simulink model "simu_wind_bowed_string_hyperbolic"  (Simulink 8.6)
settings: Solver=ode4  StartTime=0.0  StopTime=runtime  FixedStep=1/fs  RelTol=1e-3
PostLoadFcn:
  | , if any(exist('dsrtsu_mdlpostloadfcn', 'file') == [2, 3, 6]), try dsrtsu_mdlpostloadfcn('Execute', bdroot); catch fprintf('Error in PostLoadFcn (dsrtsu_mdlpostloadfcn) for model "%s":
  |  %s
  | ', bdroot, lasterr); end, end,
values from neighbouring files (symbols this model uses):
  alpha = 0.5    [bowed_string_hyperbolic.m]    (also in polynomial.m = 100)
  an = modal_coeff(:,1)    [hybrid_wind.m]
  delta = mu_d/mu_s    (= 0.375)    [bowed_string_hyperbolic.m]
  gammab_cte = 1    [bowed_string_hyperbolic.m]
  PM = 50    [bowed_string_hyperbolic.m]    (also in lip_reed.m = 20; single_reed.m = 100)
  Qn = modal_coeff(:,3)    [hybrid_wind.m]
  Ts = 25e-6    (= 2.5e-05)    [hybrid_wind.m]    (also in measurements.m)
  wn = modal_coeff(:,2)    [hybrid_wind.m]
  Zc = rho*c/St    (= 2615281.00417)    [hybrid_wind.m]
  zetab_cte = 0.2    [bowed_string_hyperbolic.m]
undefined symbols (not defined in the file or in its folder): modal_coeff, vibrato
libraries: simulink x4

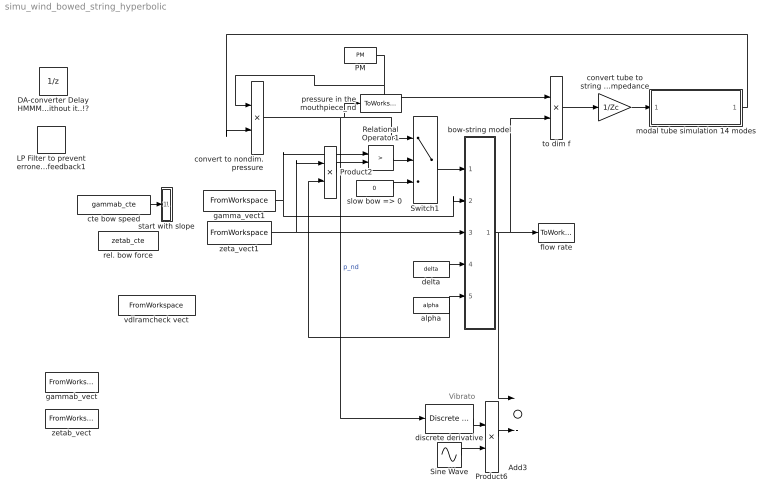
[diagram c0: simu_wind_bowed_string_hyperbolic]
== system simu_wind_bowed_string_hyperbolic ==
  note: Vibrato
  Add3 : Sum
  DA-converter Delay HMMM I don't know why this causes a less hybrid-corresponding result than without it..!? : UnitDelay  SampleTime=-1
  LP Filter to prevent erroneous high freq feedback1 : DiscreteFilter  Numerator=HdLP.ScaleValues(1)*HdLP.sosMatrix(1:end/2)  Denominator=HdLP.ScaleValues(2)*HdLP.sosMatrix(1+end/2:end)  SampleTime=Ts
  PM : Constant  Value=PM
  Product2 : Product  SampleTime=Ts
  Product6 : Product
  Relational Operator1 : RelationalOperator  Operator=>  OutDataTypeStr=boolean  SampleTime=Ts
  Sine Wave : Sin  Amplitude=vibrato.amp  Bias=-vibrato.amp  Frequency=vibrato.freq*2*pi  SampleTime=0
  Switch1 : Switch  Criteria=u2 > Threshold
  alpha : Constant  Value=alpha
  bow-string model : Subsystem
  convert tube to string characteristic impedance : Gain  Gain=1/Zc
  convert to nondim. pressure : Product  Inputs=/*
  cte bow speed : Constant  Value=gammab_cte
  delta : Constant  Value=delta
  discrete derivative : simulink/Discrete/Discrete Derivative  gainval=1.0  ICPrevScaledInput=0.0  InputProcessing=Inherited  OutMin=[]  OutMax=[]  OutDataType=fixdt(1, 16)  OutScaling=2^-10  DoSatur=off
  flow rate : ToWorkspace  VariableName=q_dl  SaveFormat=Structure  SampleTime=-1
  gamma_vect1 : FromWorkspace  VariableName=gammab_envs_all  SampleTime=0
  gammab_vect : FromWorkspace  VariableName=gammab_vect  SampleTime=Ts  OutputAfterFinalValue=Setting to zero
  modal tube simulation 14 modes : Subsystem
  pressure in the mouthpiece_nd : ToWorkspace  VariableName=p_dl  SaveFormat=Structure  SampleTime=-1
  rel. bow force : Constant  Value=zetab_cte
  slow bow => 0 : Constant  Value=0
  start with slope : Subsystem
  to dim f : Product
  vdlramcheck vect : FromWorkspace  VariableName=gammabrampcheck_vect  SampleTime=Ts  OutputAfterFinalValue=Setting to zero
  zeta_vect1 : FromWorkspace  VariableName=zetab_envs_all  SampleTime=0  OutputAfterFinalValue=Setting to zero
  zetab_vect : FromWorkspace  VariableName=zetab_vect  SampleTime=Ts  OutputAfterFinalValue=Setting to zero
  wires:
  PM/1 -> to dim f/1, convert to nondim. pressure/1
  modal tube simulation 14 modes/1(p_sim_out) -> convert to nondim. pressure/2
  delta/1 -> bow-string model/4(deltab)
  convert tube to string characteristic impedance/1 -> modal tube simulation 14 modes/1(flowrate_in)
  bow-string model/1(f) -> flow rate/1, to dim f/2, Add3/1
  to dim f/1 -> convert tube to string characteristic impedance/1
  cte bow speed/1 -> start with slope/1(gamma_in)
  convert to nondim. pressure/1 -> Switch1/1, pressure in the mouthpiece_nd/1, discrete derivative/1  "p_nd"
  discrete derivative/1 -> Product6/1
  Sine Wave/1 -> Product6/2
  Add3/1 -> ?  "new fdl"
  Product6/1 -> Add3/2
  alpha/1 -> Product2/2, bow-string model/5(alpha)
  zeta_vect1/1 -> bow-string model/3(zetab), Product2/1
  Relational Operator1/1 -> Switch1/2
  slow bow => 0/1 -> Switch1/3
  Switch1/1 -> bow-string model/1(vdl)
  Product2/1 -> Relational Operator1/2
  gamma_vect1/1 -> bow-string model/2(vbdl), Relational Operator1/1

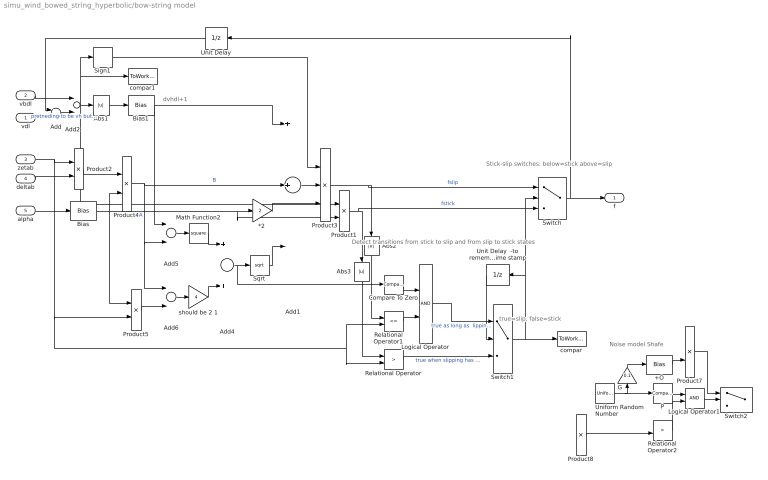
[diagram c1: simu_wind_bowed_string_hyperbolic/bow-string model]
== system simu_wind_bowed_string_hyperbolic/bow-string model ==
  note: Stick-slip switches: below=stick above=slip
  note: true=slip, false=stick
  note: dvhdl+1
  note: Detect transitions from stick to slip and from slip to stick states
  note: Noise model Shafe
  vdl : Inport
  vbdl : Inport  Port=2
  zetab : Inport  Port=3
  deltab : Inport  Port=4
  alpha : Inport  Port=5
  "*2 " : Gain  Gain=2
  +O : Bias  Bias=1
  Abs1 : Abs
  Abs2 : Abs
  Abs3 : Abs
  Add : Sum  Inputs=-+
  Add1 : Sum  Inputs=++-
  Add2 : Sum  Inputs=+-
  Add4 : Sum
  Add5 : Sum  Inputs=+-
  Add6 : Sum  Inputs=+-
  Bias : Bias  Bias=1
  Bias1 : Bias  Bias=1
  Compare To Zero : simulink/Logic and Bit Operations/Compare To Zero  relop=>  OutDataTypeStr=uint8
  G : Gain  Gain=0.1
  Logical Operator : Logic  AllPortsSameDT=off  OutDataTypeStr=boolean
  Logical Operator1 : Logic  AllPortsSameDT=off  OutDataTypeStr=boolean
  Math Function2 : Math  Operator=square
  P : simulink/Logic and Bit Operations/Compare To Constant  relop=>  const=0.5  OutDataTypeStr=uint8
  Product1 : Product  Inputs=*/
  Product{2,4..5,7..8} (5 alike) : Product
  Product3 : Product  Inputs=**/
  Relational Operator : RelationalOperator  Operator=>  OutDataTypeStr=boolean
  Relational Operator1 : RelationalOperator  Operator=<=  OutDataTypeStr=boolean
  Relational Operator2 : RelationalOperator  Operator=>  OutDataTypeStr=boolean
  Sign1 : Signum
  Sqrt : Sqrt  OutputSignalType=real
  Switch : Switch  Criteria=u2 > Threshold
  Switch1 : Switch  Criteria=u2 > Threshold
  Switch2 : Switch  Criteria=u2 > Threshold
  Uniform Random Number : UniformRandomNumber  Minimum=0  SampleTime=Ts
  Unit Delay : UnitDelay  SampleTime=-1
  Unit Delay  -to remember slip/stick state of previous time stamp : UnitDelay  SampleTime=-1
  compar : ToWorkspace  VariableName=compar  SaveFormat=Structure  SampleTime=-1
  compar1 : ToWorkspace  VariableName=dvhdl  SaveFormat=Structure  SampleTime=-1
  should be 2 1 : Gain  Gain=4
  f : Outport
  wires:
  vbdl/1 -> Add2/1
  Switch1/1 -> Switch/2, Unit Delay  -to remember slip/stick state of previous time stamp/1, compar/1
  Unit Delay  -to remember slip/stick state of previous time stamp/1 -> Switch1/2
  Add2/1 -> Abs1/1, Product1/1, Sign1/1, compar1/1
  Relational Operator/1 -> Switch1/3  "true when slipping has to start"
  Unit Delay/1 -> Add/1
  Add/1 -> Add2/2  "pretneding to be vh but is actually vh-1"
  vdl/1 -> Add/2
  Logical Operator/1 -> Switch1/1  "true as long as  lipping is happening"
  zetab/1 -> Product2/1, Product5/2, Relational Operator1/2, Relational Operator/2
  deltab/1 -> Product2/2
  Product2/1 -> Product4/1
  alpha/1 -> Bias/1
  Bias/1 -> Product1/2, "*2 "/1, Product5/1, Product4/2  "A"
  Product4/1 -> Add1/2, Add5/2, Add6/1  "B"
  Bias1/1 -> Add1/1, Add5/1
  Sqrt/1 -> Add1/3
  Add4/1 -> Sqrt/1, Compare To Zero/1
  Math Function2/1 -> Add4/1
  Add6/1 -> should be 2 1/1
  Add5/1 -> Math Function2/1
  should be 2 1/1 -> Add4/2
  Product5/1 -> Add6/2
  Abs1/1 -> Bias1/1
  Sign1/1 -> Product3/1
  Add1/1 -> Product3/2
  "*2 "/1 -> Product3/3
  Product1/1 -> Switch/3, Abs3/1  "fstick"
  Product3/1 -> Switch/1, Abs2/1  "fslip"
  Compare To Zero/1 -> Logical Operator/1
  Relational Operator1/1 -> Logical Operator/2
  Switch/1 -> Unit Delay/1, f/1
  Abs2/1 -> Relational Operator1/1
  Abs3/1 -> Relational Operator/1
  Logical Operator1/1 -> Switch2/2
  P/1 -> Logical Operator1/1
  Relational Operator2/1 -> Logical Operator1/2
  Uniform Random Number/1 -> P/1, G/1
  G/1 -> +O/1
  +O/1 -> Product7/2
  Product7/1 -> Switch2/1
  ? -> Relational Operator2/1  "dvhdl"
  Product8/1 -> Relational Operator2/2
  ? -> Product8/1  "1+alpha"
  ? -> Product8/2  "zetab"
  ? -> Product7/1  "fdl in"
  Switch2/1 -> ?  "fdl out"
  ? -> Switch2/3  "fdl in"

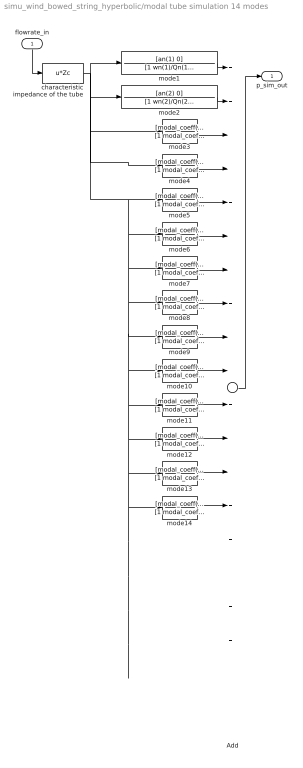
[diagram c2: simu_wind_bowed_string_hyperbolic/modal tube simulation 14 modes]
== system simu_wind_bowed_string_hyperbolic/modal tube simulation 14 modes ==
  flowrate_in : Inport
  Add : Sum  Inputs=++++++++++++++++++++
  characteristic impedance of the tube : Fcn  Expr=u*Zc
  mode1 : TransferFcn  Numerator=[an(1) 0]  Denominator=[1 wn(1)/Qn(1) wn(1)^2]
  mode10 : TransferFcn  Numerator=[modal_coeff(10, 1) 0]  Denominator=[1 modal_coeff(10,2)/modal_coeff(10,3) modal_coeff(10,2)^2]
  mode11 : TransferFcn  Numerator=[modal_coeff(11, 1) 0]  Denominator=[1 modal_coeff(11,2)/modal_coeff(11,3) modal_coeff(11,2)^2]
  mode12 : TransferFcn  Numerator=[modal_coeff(12, 1) 0]  Denominator=[1 modal_coeff(12,2)/modal_coeff(12,3) modal_coeff(12,2)^2]
  mode13 : TransferFcn  Numerator=[modal_coeff(13, 1) 0]  Denominator=[1 modal_coeff(13,2)/modal_coeff(13,3) modal_coeff(13,2)^2]
  mode14 : TransferFcn  Numerator=[modal_coeff(14, 1) 0]  Denominator=[1 modal_coeff(14,2)/modal_coeff(14,3) modal_coeff(14,2)^2]
  mode2 : TransferFcn  Numerator=[an(2) 0]  Denominator=[1 wn(2)/Qn(2) wn(2)^2]
  mode3 : TransferFcn  Numerator=[modal_coeff(3, 1) 0]  Denominator=[1 modal_coeff(3,2)/modal_coeff(3,3) modal_coeff(3,2)^2]
  mode4 : TransferFcn  Numerator=[modal_coeff(4, 1) 0]  Denominator=[1 modal_coeff(4,2)/modal_coeff(4,3) modal_coeff(4,2)^2]
  mode5 : TransferFcn  Numerator=[modal_coeff(5, 1) 0]  Denominator=[1 modal_coeff(5,2)/modal_coeff(5,3) modal_coeff(5,2)^2]
  mode6 : TransferFcn  Numerator=[modal_coeff(6, 1) 0]  Denominator=[1 modal_coeff(6,2)/modal_coeff(6,3) modal_coeff(6,2)^2]
  mode7 : TransferFcn  Numerator=[modal_coeff(7, 1) 0]  Denominator=[1 modal_coeff(7,2)/modal_coeff(7,3) modal_coeff(7,2)^2]
  mode8 : TransferFcn  Numerator=[modal_coeff(8, 1) 0]  Denominator=[1 modal_coeff(8,2)/modal_coeff(8,3) modal_coeff(8,2)^2]
  mode9 : TransferFcn  Numerator=[modal_coeff(9, 1) 0]  Denominator=[1 modal_coeff(9,2)/modal_coeff(9,3) modal_coeff(9,2)^2]
  p_sim_out : Outport
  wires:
  flowrate_in/1 -> characteristic impedance of the tube/1
  characteristic impedance of the tube/1 -> mode4/1, mode3/1, mode2/1, mode1/1, mode5/1, mode6/1, mode7/1, mode8/1, mode9/1, mode10/1, mode11/1, mode12/1, mode13/1, mode14/1
  mode1/1 -> Add/1
  Add/1 -> p_sim_out/1
  mode2/1 -> Add/2
  mode3/1 -> Add/3
  mode4/1 -> Add/4
  mode5/1 -> Add/5
  mode6/1 -> Add/6
  mode7/1 -> Add/7
  mode8/1 -> Add/8
  mode9/1 -> Add/9
  mode10/1 -> Add/10
  mode11/1 -> Add/11
  mode12/1 -> Add/12
  mode13/1 -> Add/13
  ? -> Add/15
  mode14/1 -> Add/14

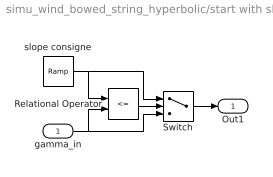
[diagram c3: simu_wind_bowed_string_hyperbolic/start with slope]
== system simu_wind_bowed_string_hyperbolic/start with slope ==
  gamma_in : Inport
  Relational Operator : RelationalOperator  Operator=<=  OutDataTypeStr=boolean
  Switch : Switch  Criteria=u2 > Threshold
  slope consigne : simulink/Sources/Ramp  slope=gammab_cte*100  start=0  X0=0
  Out1 : Outport
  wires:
  slope consigne/1 -> Relational Operator/1, Switch/1
  gamma_in/1 -> Relational Operator/2, Switch/3
  Relational Operator/1 -> Switch/2
  Switch/1 -> Out1/1
